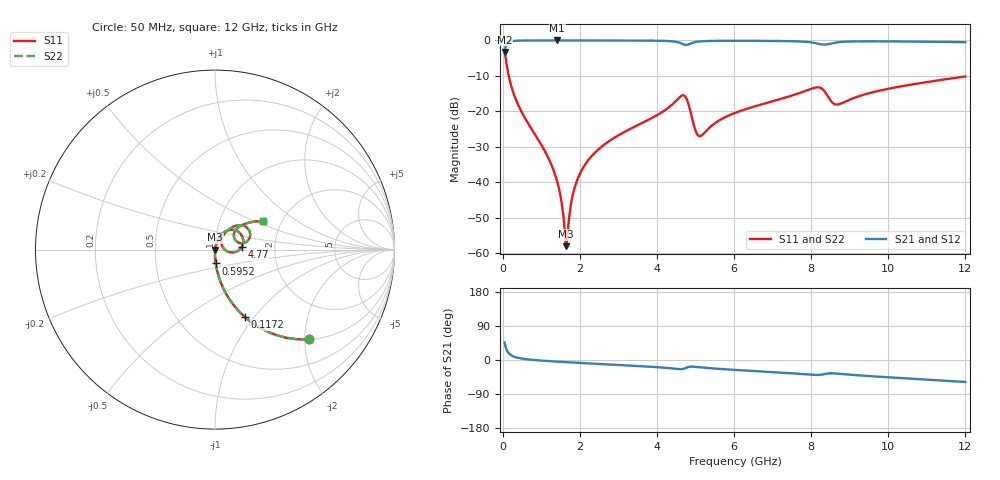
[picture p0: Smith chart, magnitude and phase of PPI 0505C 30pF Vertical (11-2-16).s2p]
# GHz S MA R 50
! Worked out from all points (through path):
!   1601 points, 50 MHz to 12 GHz, reference 50 ohm
!   highest |S21| = -0.01 dB at 1.417 GHz (marker M1); lowest = -3.3 dB at 50 MHz (marker M2)
!   group delay of S21, straight-line fit = 14.1 ps
!   lowest |S11| = -58.1 dB at 1.648 GHz (marker M3), VSWR 1.00, Z = 50.1 - j0.0188 ohm
!   |S11| at or under -10 dB: 157.2 MHz to end of sweep
!   |S22| runs from -58.1 to -2.8 dB; largest |S21 - S12| = 0
!   S11 on the Smith chart (normalised r, x): 50 MHz: 0.99, -2.11; 117.2 MHz: 0.99, -0.89; 595.2 MHz: 1.00, -0.15; 4.77 GHz: 1.35, +0.04; 12 GHz: 1.60, +0.56
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0.05  0.7262 -43.6  0.6873 46.4  0.6873 46.4  0.7262 -43.6
0.1172187  0.4094 -66.2  0.912 23.8  0.912 23.8  0.4094 -66.2
0.2964688  0.1701 -81.0  0.9848 8.8  0.9848 8.8  0.1701 -81.0
0.5952188  0.07728 -87.1  0.9962 2.4  0.9962 2.4  0.07728 -87.1
1.147906  0.0241 -90.1  0.9986 -2.6  0.9986 -2.6  0.0241 -90.1
1.416781  0.01008 -87.7  0.9987 -4.3  0.9987 -4.3  0.01008 -87.7
1.648313  0.00125 -8.6  0.9986 -5.7  0.9986 -5.7  0.00125 -8.6
1.685656  0.001898 42.3  0.9986 -5.9  0.9986 -5.9  0.001898 42.3
1.835031  0.007208 72.7  0.9985 -6.8  0.9985 -6.8  0.007208 72.7
2.044156  0.01457 76.5  0.9984 -7.9  0.9984 -7.9  0.01457 76.5
2.671531  0.03508 75.9  0.9975 -11.3  0.9975 -11.3  0.03508 75.9
4.038312  0.09046 66.8  0.9893 -19.1  0.9893 -19.1  0.09046 66.8
4.635813  0.1653 34.9  0.9045 -24.1  0.9045 -24.1  0.1653 34.9
4.77025  0.1496 5.6  0.8629 -20.2  0.8629 -20.2  0.1496 5.6
4.994313  0.05476 -0.7  0.9473 -18.1  0.9473 -18.1  0.05476 -0.7
5.098875  0.04467 22.6  0.9659 -19.2  0.9659 -19.2  0.04467 22.6
6.025  0.09483 59.5  0.9878 -26.1  0.9878 -26.1  0.09483 59.5
8.019156  0.2096 38.8  0.9341 -39.1  0.9341 -39.1  0.2096 38.8
8.265625  0.2109 21.7  0.8783 -38.6  0.8783 -38.6  0.2109 21.7
8.668938  0.1246 28.4  0.939 -35.8  0.939 -35.8  0.1246 28.4
10.01331  0.2084 41.8  0.9683 -45.7  0.9683 -45.7  0.2084 41.8
12  0.3098 30.8  0.9433 -58.0  0.9433 -58.0  0.3098 30.8
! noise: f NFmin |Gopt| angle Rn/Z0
0.05  0.0003886  0.865  0.8153  0.000618
1.372  0.004  0.6752  4.815  0.002371
2.701  0.006954  0.6408  9.145  0.003635
4.031  0.01595  0.7519  13.7  0.01278
5.36  0.02894  0.8131  18.35  0.0315
6.682  0.02102  0.7017  22.39  0.0133
8.012  0.05926  0.8625  27.09  0.08739
9.341  0.03663  0.7582  31.15  0.0285
10.67  0.02855  0.6687  34.58  0.01516
12  0.02889  0.6435  38.03  0.01378
